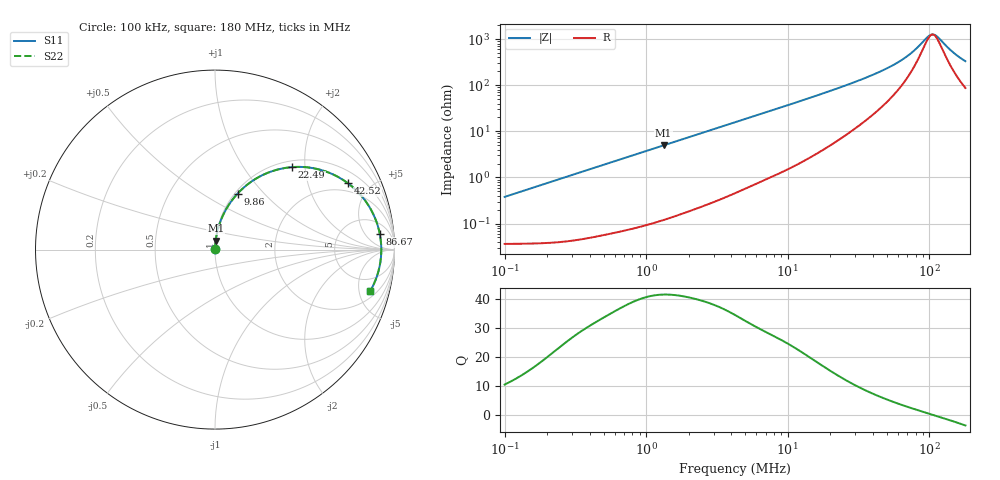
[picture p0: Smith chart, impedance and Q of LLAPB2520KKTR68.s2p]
! LLAPB2520KKTR68  S-PARAMETER MODEL  ( General Type )
! Model Generated by TAIYO YUDEN Corporation (http://www.ty-top.com)
! Version 2.0
! TAIYO YUDEN Control No. 20210629
! Copyright(c) 2015 TAIYO YUDEN CO.,LTD. All Rights Reserved.
! Product Description (link to TY-COMPAS)
! https://ds.yuden.co.jp/TYCOMPAS/or/detail?pn=LLAPB2520KKTR68M&u=M
! Products Name : Inductors
! Characteristics :
!  Inductance : 0.68 uH , SRF(min) : -Hz , DC Resistance(max) : 0.043 Ohm
!  Rated Current : Saturation :4300 mA , Temp Rise : 3400 mA (40 degC)
!  Case Size : 2.5 x 2.0 / 0.098 x 0.079 [mm/inch] , Thickness : 1 / 0.039 [mm/inch]
!  (Conditions: Temperature = 25 degC , DC Bias Current/Voltage = 0A / 0V)
! External Node Assignments :
!  1  o---GGG---o  2
! GND o---------o GND
! Frequency Range : 0.1MHz  -  180.004543MHz  [ 402 STEP ]
# MHz S RI R 50
! Freq[MHz].  S11 Real  S11 Imag  S21 Real  S21 Imag  S12 Real  S12 Imag  S22 Real  S22 Imag
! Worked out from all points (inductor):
!   401 points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, 100 kHz to 180 MHz, reference 50 ohm
!   read as one part in series: L = 601 nH near 103.8 kHz
!   highest Q = 41.5 at 1.328 MHz (marker M1), where L = 594 nH
!   self-resonance near 105.6 MHz
!   S11 on the Smith chart (normalised r, x): 100 kHz: 1.00, +0.01; 9.86 MHz: 1.03, +0.73; 22.49 MHz: 1.13, +1.71; 42.52 MHz: 1.54, +3.61; 86.67 MHz: 10, +12; 180 MHz: 2.74, -6.40
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0.1  0.000376 0.00377  0.9996 -0.00377  0.9996 -0.00377  0.000376 0.00377
0.350962  0.000633 0.0132  0.9994 -0.0132  0.9994 -0.0132  0.000633 0.0132
1.231743  0.00322 0.0458  0.9968 -0.0458  0.9968 -0.0458  0.00322 0.0458
1.327617  0.00364 0.0493  0.9964 -0.0493  0.9964 -0.0493  0.00364 0.0493
2.510567  0.0109 0.0919  0.9891 -0.0919  0.9891 -0.0919  0.0109 0.0919
4.322947  0.0291 0.1542  0.9709 -0.1542  0.9709 -0.1542  0.0291 0.1542
6.777928  0.0656 0.2309  0.9344 -0.2309  0.9344 -0.2309  0.0656 0.2309
9.859641  0.1261 0.3124  0.8739 -0.3124  0.8739 -0.3124  0.1261 0.3124
14.89024  0.2454 0.4051  0.7546 -0.4051  0.7546 -0.4051  0.2454 0.4051
22.48756  0.4278 0.4594  0.5722 -0.4594  0.5722 -0.4594  0.4278 0.4594
30.92373  0.5911 0.4435  0.4089 -0.4435  0.4089 -0.4435  0.5911 0.4435
42.52471  0.7397 0.3705  0.2603 -0.3705  0.2603 -0.3705  0.7397 0.3705
52.25907  0.8156 0.2998  0.1844 -0.2998  0.1844 -0.2998  0.8156 0.2998
69.22052  0.8872 0.186  0.1128 -0.186  0.1128 -0.186  0.8872 0.186
77.45761  0.9055 0.1374  0.0945 -0.1374  0.0945 -0.1374  0.9055 0.1374
86.6749  0.918 0.0879  0.082 -0.0879  0.082 -0.0879  0.918 0.0879
98.82363  0.9255 0.0296  0.0745 -0.0296  0.0745 -0.0296  0.9255 0.0296
104.5383  0.9265 0.00447  0.0735 -0.00447  0.0735 -0.00447  0.9265 0.00447
108.5305  0.9264 -0.0123  0.0736 0.0123  0.0736 0.0123  0.9264 -0.0123
114.8065  0.9251 -0.0374  0.0749 0.0374  0.0749 0.0374  0.9251 -0.0374
149.2455  0.9005 -0.1533  0.0995 0.1533  0.0995 0.1533  0.9005 -0.1533
180.0045  0.8638 -0.233  0.1362 0.233  0.1362 0.233  0.8638 -0.233
